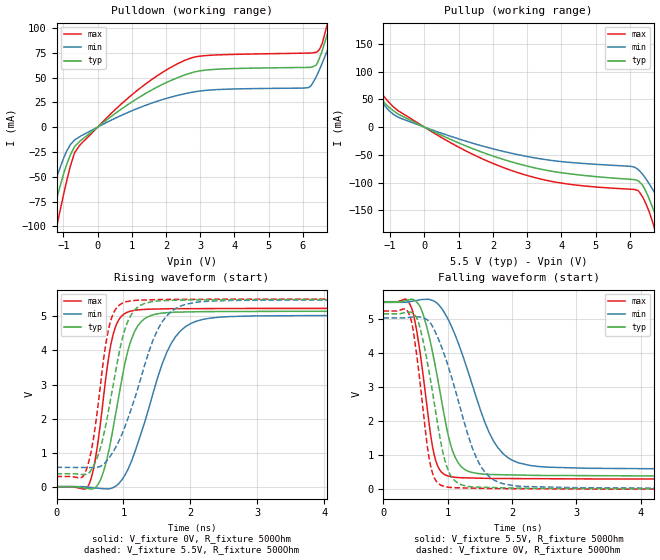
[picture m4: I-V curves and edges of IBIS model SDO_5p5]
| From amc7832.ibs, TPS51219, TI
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|   Model
[Model]   SDO_5p5
Model_type   Output
Polarity   Non-Inverting
Vmeas = 2.75
Vref = 0
Cref = 1pF
Rref = 100000
|   typ   min   max
C_comp   1pF   1pF   1pF
[Voltage Range]   5.5   5.49   5.51
[Temperature Range]   27   125   -40
[Pullup Reference]   5.5   5.49   5.51
[Pulldown Reference]   -0   -0   -0
[Power Clamp Reference]   5.5   5.49   5.51
[GND Clamp Reference]   -0   -0   -0
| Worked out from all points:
|   slope of the pulldown table from 0 to 0.825 V, typ, clamps not added: 38.8 ohm
|   slope of the pullup table from 0 to 0.825 V, typ, clamps not added: 34.7 ohm
|   falling waveform, V_fixture 5.5V, R_fixture 500Ohm: 20-80 % time 320ps typ, 553ps min, 222ps max; typ from 5.5 V to 0.378 V
|   rising waveform, V_fixture 0V, R_fixture 500Ohm: 20-80 % time 308ps typ, 500ps min, 214ps max; typ from 0 V to 5.16 V
|   rising waveform, V_fixture 5.5V, R_fixture 500Ohm: 20-80 % time 310ps typ, 507ps min, 215ps max; typ from 0.378 V to 5.5 V
|   falling waveform, V_fixture 0V, R_fixture 500Ohm: 20-80 % time 288ps typ, 493ps min, 200ps max; typ from 5.16 V to 0 V
[Pulldown]
|   Voltage   I(typ)   I(min)   I(max)
-5.5V     -888.8mA   -641.4mA   -1.134A
-2.563V   -320.5mA   -219.9mA   -419mA
-1.375V   -101.7mA   -69.84mA   -135.7mA
-1.226V   -77.61mA   -53.82mA   -105.8mA
-797.5mV  -28.13mA   -17.73mA   -39.54mA
-517mV    -14.13mA   -9.502mA   -18.02mA
2.552V    52.69mA    33.72mA    67.43mA
6.165V    60.23mA    39.92mA    74.67mA
6.479V    69.03mA    57.65mA    77.95mA
6.71V     93.12mA    76.91mA    103.4mA
7.106V    139.1mA    112mA      161.6mA
10.98V    365.3mA    303mA      431mA
[Pullup]
|   Voltage   I(typ)   I(min)   I(max)
-5.5V     297.6mA    253.2mA    343.1mA
-3.586V   226mA      191.8mA    260.5mA
-2.794V   186mA      157.1mA    216.5mA
-2.183V   142.5mA    120.6mA    167.2mA
-1.375V   62.1mA     56.22mA    71.11mA
-764.5mV  23.41mA    17.92mA    29.35mA
2.717V    -65.64mA   -49.42mA   -81.75mA
6.231V    -96.32mA   -75.68mA   -114.2mA
6.726V    -154.4mA   -118.4mA   -183.6mA
6.891V    -182.4mA   -136.5mA   -220.9mA
8.079V    -403.7mA   -288.3mA   -507.7mA
10.98V    -970mA     -708.5mA   -1.218A
[Ramp]
R_load = 500
|   typ   min   max
dV/dt_r   3.09283/3.0787e-10   3.02016/4.99762e-10   3.14221/2.14273e-10
dV/dt_f   3.07306/3.19539e-10   2.95351/5.53101e-10   3.12777/2.2154e-10
[Falling Waveform]
V_fixture = 5.5V
V_fixture_min = 5.49V
V_fixture_max = 5.51V
R_fixture = 500Ohm
C_fixture = 0F
|   Time   V(typ)   V(min)   V(max)
0s        5.5V       5.49V      5.51V
386.3ps   5.562V     5.506V     5.517V
468.7ps   5.569V     5.533V     5.133V
574ps     5.351V     5.567V     3.962V
733.4ps   4.297V     5.566V     1.599V
816.6ps   3.515V     5.493V     816.9mV
1.096ns   1.024V     4.617V     352.8mV
1.711ns   429.2mV    1.414V     314.3mV
2.41ns    404.3mV    666.8mV    308mV
20ns      378.2mV    567.5mV    297.1mV
[Rising Waveform]
V_fixture = 0V
V_fixture_min = 0V
V_fixture_max = 0V
R_fixture = 500Ohm
C_fixture = 0F
|   Time   V(typ)   V(min)   V(max)
0s        351.3nV    -1.362uV   -11.67nV
452.5ps   -50.55mV   -11.06mV   -38.14mV
644.8ps   151.1mV    -50.86mV   1.684V
761.1ps   879.9mV    -65.57mV   3.56V
872ps     2.01V      -1.318mV   4.645V
1.042ns   3.792V     409.6mV    5.108V
1.213ns   4.721V     1.265V     5.191V
1.711ns   5.118V     4.199V     5.226V
2.41ns    5.143V     4.974V     5.231V
20ns      5.155V     5.034V     5.237V
[Rising Waveform]
V_fixture = 5.5V
V_fixture_min = 5.49V
V_fixture_max = 5.51V
R_fixture = 500Ohm
C_fixture = 0F
|   Time   V(typ)   V(min)   V(max)
0s        378.2mV    567.4mV    297.1mV
399.6ps   355.3mV    561.3mV    307.7mV
501.2ps   443.2mV    559.8mV    886.5mV
574ps     687.5mV    559.2mV    1.701V
788.9ps   2.362V     855mV      4.727V
951.1ps   4.081V     1.419V     5.351V
1.096ns   4.978V     2.168V     5.453V
1.578ns   5.463V     4.841V     5.498V
2.181ns   5.486V     5.436V     5.504V
20ns      5.5V       5.49V      5.51V
[Falling Waveform]
|Gnd
V_fixture = 0V
V_fixture_min = 0V
V_fixture_max = 0V
R_fixture = 500Ohm
C_fixture = 0F
|   Time   V(typ)   V(min)   V(max)
0s        5.155V     5.034V     5.237V
373.1ps   5.203V     5.046V     5.241V
439.3ps   5.197V     5.059V     4.908V
523.4ps   5.009V     5.066V     3.853V
733.4ps   3.192V     4.873V     685.2mV
890.7ps   1.387V     4.246V     119.8mV
1.006ns   561.3mV    3.621V     58.15mV
1.512ns   56.71mV    675.8mV    24.64mV
2.02ns    32.53mV    103mV      13.97mV
20ns      -13.91uV   189uV      550.9nV
